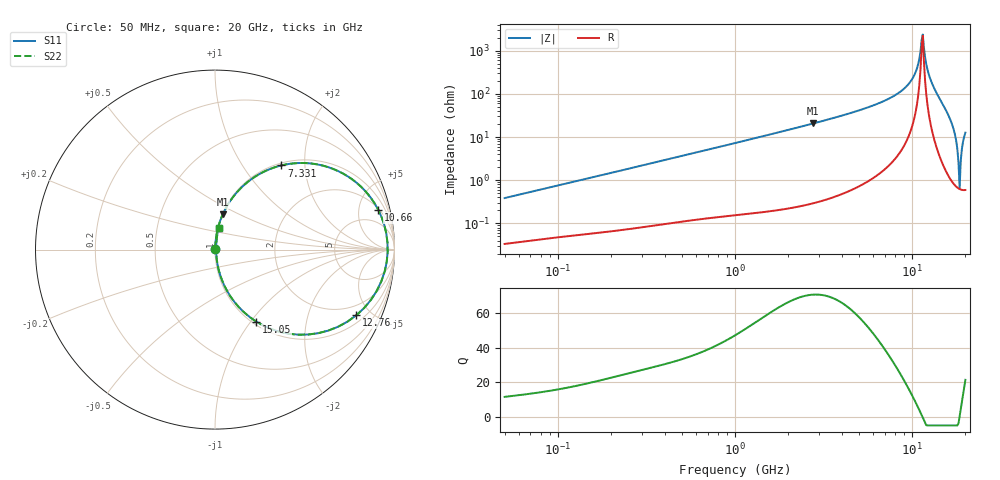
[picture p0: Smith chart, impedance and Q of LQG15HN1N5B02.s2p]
!Murata Part Number: LQG15HN1N5B02
!These Parameters are Measured in Series Mode Connection
!  o--[Z]--o
!Port1  Port2
!  o-------o
!Freq. Start=50[MHz] Stop=20[GHz], 401[Steps]
# Hz S RI R 50
!Freq.(Hz) S11(Real) S11(Imag) S21(Real) S21(Imag) S12(Real) S12(Imag) S22(Real) S22(Imag)
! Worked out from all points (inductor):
!   401 points, 50 MHz to 20 GHz, reference 50 ohm
!   read as one part in series: L = 1.21 nH near 51.52 MHz
!   highest Q = 70.6 at 2.769 GHz (marker M1), where L = 1.19 nH
!   self-resonance near 11.32 GHz
!   S11 on the Smith chart (normalised r, x): 50 MHz: 1.00, +0.01; 7.331 GHz: 1.04, +1.52; 10.66 GHz: 2.16, +7.75; 12.76 GHz: 1.37, -4.08; 15.05 GHz: 1.04, -1.06; 20 GHz: 1.01, +0.25
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5e7  0.000349 0.00384  0.9997 -0.00384  0.9997 -0.00384  0.000349 0.00384
1.364002e8  0.00065 0.0101  0.9993 -0.0101  0.9993 -0.0101  0.00065 0.0101
3.721004e8  0.00166 0.0271  0.9983 -0.0271  0.9983 -0.0271  0.00166 0.0271
1e9  0.00672 0.0718  0.9933 -0.0718  0.9933 -0.0718  0.00672 0.0718
2.728004e9  0.0421 0.1939  0.9579 -0.1939  0.9579 -0.1939  0.0421 0.1939
2.769174e9  0.0434 0.1968  0.9566 -0.1968  0.9566 -0.1968  0.0434 0.1968
5.041459e9  0.1525 0.3508  0.8475 -0.3508  0.8475 -0.3508  0.1525 0.3508
7.331367e9  0.3695 0.469  0.6305 -0.469  0.6305 -0.469  0.3695 0.469
7.442007e9  0.3838 0.4722  0.6162 -0.4722  0.6162 -0.4722  0.3838 0.4722
9.457416e9  0.7104 0.4253  0.2896 -0.4253  0.2896 -0.4253  0.7104 0.4253
1.066139e10  0.9099 0.2213  0.0901 -0.2213  0.0901 -0.2213  0.9099 0.2213
1.115139e10  0.9546 0.089  0.0454 -0.089  0.0454 -0.089  0.9546 0.089
1.149051e10  0.9619 -0.0138  0.0381 0.0138  0.0381 0.0138  0.9619 -0.0138
1.276073e10  0.7869 -0.3663  0.2131 0.3663  0.2131 0.3663  0.7869 -0.3663
1.504638e10  0.23 -0.4013  0.77 0.4013  0.77 0.4013  0.23 -0.4013
1.696185e10  0.0383 -0.1687  0.9617 0.1687  0.9617 0.1687  0.0383 -0.1687
1.747767e10  0.0197 -0.1092  0.9803 0.1092  0.9803 0.1092  0.0197 -0.1092
1.800918e10  0.00944 -0.0521  0.9906 0.0521  0.9906 0.0521  0.00944 -0.0521
1.855685e10  0.0062 0.00202  0.9938 -0.00202  0.9938 -0.00202  0.0062 0.00202
1.912117e10  0.00875 0.0529  0.9913 -0.0529  0.9913 -0.0529  0.00875 0.0529
1.940974e10  0.0119 0.0771  0.9881 -0.0771  0.9881 -0.0771  0.0119 0.0771
2e10  0.0213 0.123  0.9787 -0.123  0.9787 -0.123  0.0213 0.123
